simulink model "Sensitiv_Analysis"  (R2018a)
settings: Solver=ode4  StartTime=0.0  StopTime=40000  FixedStep=Ts  MaxStep=0.5  RelTol=1e-3  EnableMultiTasking=on
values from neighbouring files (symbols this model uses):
  Int_IC = [qti', 0 0, h0i(1:3)', 0 0, wr0, Vec0'*M0, Pec0']    [run.m]
  Kq1 = I22*ww^2 - 3*wo2*(I11-I33)    [run.m]
  Kq2 = 2*I22*zet*ww    [run.m]
  Kqi = 0.0005    [run.m]
  Kr1 = (0.1*I11*I33*zet^2/Hy0) - sqrt( ((0.01^zet^4*I11^2*I33^2)/Hy0^2)+(4*I11*I33*zet^2) )    [run.m]
  Kr2 = 0.05*Kr1    [run.m]
  Kr3 = 0.04*zet*(Kr2-Hy0) * sqrt(abs(Hy0/(I11*I33)))    [run.m]
  nt = 7    [run.m]    (also in runf.m)
  r2d = 180/pi    (= 57.2957795131)    [pl.m]    (also in pl2.m; run.m; plf.m; runf.m)
  Ts = 0.001    [run.m]    (also in runf.m = 0.0005)
undefined symbols (not defined in the file or in its folder): Aflx, Bflx, Cflx, den, Dflx, DiscIntNeverNeededParam, num, RW_Steering, Vehi_3B3W
libraries: simulink x3

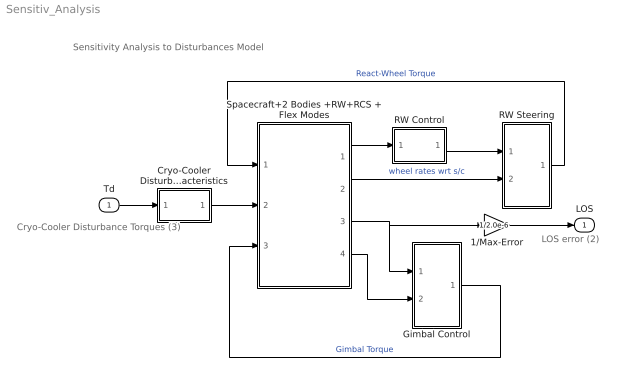
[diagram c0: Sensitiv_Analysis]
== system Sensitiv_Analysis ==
  note: Sensitivity Analysis to Disturbances Model
  note: LOS error (2)
  note: Cryo-Cooler Disturbance Torques (3)
  Td : Inport
  1/Max-Error : Gain  Gain=1/2.0e-6
  Cryo-Cooler Disturbance Characteristics : Subsystem
  Gimbal Control : Subsystem
  RW Control : Subsystem
  RW Steering : Subsystem
  Spacecraft+2 Bodies +RW+RCS + Flex Modes : Subsystem
  LOS : Outport
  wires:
  Spacecraft+2 Bodies +RW+RCS + Flex Modes/1(atti) -> RW Control/1(atti)
  Gimbal Control/1(GTrq) -> Spacecraft+2 Bodies +RW+RCS + Flex Modes/3(Tgimb)  "Gimbal Torque"
  RW Control/1(Tc) -> RW Steering/1(Trwc)
  Spacecraft+2 Bodies +RW+RCS + Flex Modes/2(Wrw) -> RW Steering/2(wr(1))  "wheel rates wrt s/c"
  RW Steering/1(Twi) -> Spacecraft+2 Bodies +RW+RCS + Flex Modes/1(Trw)  "React-Wheel Torque"
  Td/1 -> Cryo-Cooler Disturbance Characteristics/1(in)
  Spacecraft+2 Bodies +RW+RCS + Flex Modes/3(gimb) -> Gimbal Control/1(Gimb), 1/Max-Error/1
  Cryo-Cooler Disturbance Characteristics/1(ou) -> Spacecraft+2 Bodies +RW+RCS + Flex Modes/2(Tdist)
  1/Max-Error/1 -> LOS/1
  Spacecraft+2 Bodies +RW+RCS + Flex Modes/4(Gmb-dot) -> Gimbal Control/2(Grat)

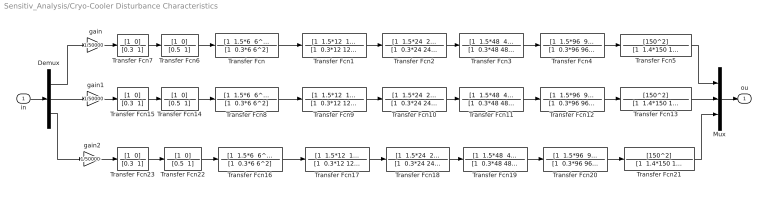
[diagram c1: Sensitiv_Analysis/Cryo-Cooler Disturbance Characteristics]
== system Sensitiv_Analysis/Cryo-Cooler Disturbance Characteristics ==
  in : Inport
  Demux : Demux  Outputs=3
  Mux : Mux  Inputs=3
  Transfer Fcn : TransferFcn  Numerator="[1  1.5*6  6^2]"  Denominator="[1  0.3*6 6^2]"
  Transfer Fcn1 : TransferFcn  Numerator="[1  1.5*12  12^2]"  Denominator="[1  0.3*12 12^2]"
  Transfer Fcn10 : TransferFcn  Numerator="[1  1.5*24  24^2]"  Denominator="[1  0.3*24 24^2]"
  Transfer Fcn11 : TransferFcn  Numerator="[1  1.5*48  48^2]"  Denominator="[1  0.3*48 48^2]"
  Transfer Fcn12 : TransferFcn  Numerator="[1  1.5*96  96^2]"  Denominator="[1  0.3*96 96^2]"
  Transfer Fcn13 : TransferFcn  Numerator=[150^2]  Denominator="[1  1.4*150 150^2]"
  Transfer Fcn14 : TransferFcn  Numerator="[1  0]"  Denominator="[0.5  1]"
  Transfer Fcn15 : TransferFcn  Numerator="[1  0]"  Denominator="[0.3  1]"
  Transfer Fcn16 : TransferFcn  Numerator="[1  1.5*6  6^2]"  Denominator="[1  0.3*6 6^2]"
  Transfer Fcn17 : TransferFcn  Numerator="[1  1.5*12  12^2]"  Denominator="[1  0.3*12 12^2]"
  Transfer Fcn18 : TransferFcn  Numerator="[1  1.5*24  24^2]"  Denominator="[1  0.3*24 24^2]"
  Transfer Fcn19 : TransferFcn  Numerator="[1  1.5*48  48^2]"  Denominator="[1  0.3*48 48^2]"
  Transfer Fcn2 : TransferFcn  Numerator="[1  1.5*24  24^2]"  Denominator="[1  0.3*24 24^2]"
  Transfer Fcn20 : TransferFcn  Numerator="[1  1.5*96  96^2]"  Denominator="[1  0.3*96 96^2]"
  Transfer Fcn21 : TransferFcn  Numerator=[150^2]  Denominator="[1  1.4*150 150^2]"
  Transfer Fcn22 : TransferFcn  Numerator="[1  0]"  Denominator="[0.5  1]"
  Transfer Fcn23 : TransferFcn  Numerator="[1  0]"  Denominator="[0.3  1]"
  Transfer Fcn3 : TransferFcn  Numerator="[1  1.5*48  48^2]"  Denominator="[1  0.3*48 48^2]"
  Transfer Fcn4 : TransferFcn  Numerator="[1  1.5*96  96^2]"  Denominator="[1  0.3*96 96^2]"
  Transfer Fcn5 : TransferFcn  Numerator=[150^2]  Denominator="[1  1.4*150 150^2]"
  Transfer Fcn6 : TransferFcn  Numerator="[1  0]"  Denominator="[0.5  1]"
  Transfer Fcn7 : TransferFcn  Numerator="[1  0]"  Denominator="[0.3  1]"
  Transfer Fcn8 : TransferFcn  Numerator="[1  1.5*6  6^2]"  Denominator="[1  0.3*6 6^2]"
  Transfer Fcn9 : TransferFcn  Numerator="[1  1.5*12  12^2]"  Denominator="[1  0.3*12 12^2]"
  gain : Gain  Gain=1/50000
  gain1 : Gain  Gain=1/50000
  gain2 : Gain  Gain=1/50000
  ou : Outport
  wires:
  Demux/1 -> gain/1
  Transfer Fcn/1 -> Transfer Fcn1/1
  Transfer Fcn1/1 -> Transfer Fcn2/1
  Transfer Fcn2/1 -> Transfer Fcn3/1
  Transfer Fcn3/1 -> Transfer Fcn4/1
  gain/1 -> Transfer Fcn7/1
  Transfer Fcn4/1 -> Transfer Fcn5/1
  Transfer Fcn5/1 -> Mux/1
  Transfer Fcn6/1 -> Transfer Fcn/1
  Transfer Fcn7/1 -> Transfer Fcn6/1
  Demux/2 -> gain1/1
  Transfer Fcn8/1 -> Transfer Fcn9/1
  Transfer Fcn9/1 -> Transfer Fcn10/1
  Transfer Fcn10/1 -> Transfer Fcn11/1
  Transfer Fcn11/1 -> Transfer Fcn12/1
  gain1/1 -> Transfer Fcn15/1
  Transfer Fcn12/1 -> Transfer Fcn13/1
  Transfer Fcn13/1 -> Mux/2
  Transfer Fcn14/1 -> Transfer Fcn8/1
  Transfer Fcn15/1 -> Transfer Fcn14/1
  Demux/3 -> gain2/1
  Transfer Fcn16/1 -> Transfer Fcn17/1
  Transfer Fcn17/1 -> Transfer Fcn18/1
  Transfer Fcn18/1 -> Transfer Fcn19/1
  Transfer Fcn19/1 -> Transfer Fcn20/1
  gain2/1 -> Transfer Fcn23/1
  Transfer Fcn20/1 -> Transfer Fcn21/1
  Transfer Fcn21/1 -> Mux/3
  Transfer Fcn22/1 -> Transfer Fcn16/1
  Transfer Fcn23/1 -> Transfer Fcn22/1
  Mux/1 -> ou/1
  in/1 -> Demux/1

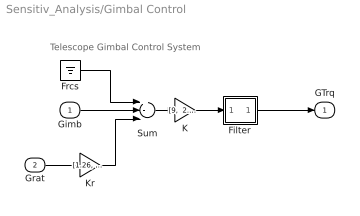
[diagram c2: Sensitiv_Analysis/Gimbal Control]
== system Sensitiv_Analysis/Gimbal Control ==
  note: Telescope Gimbal Control System
  Gimb : Inport
  Grat : Inport  Port=2
  Filter : Subsystem
  Frcs : Ground
  K : Gain  Gain="[9,  2.85]"
  Kr : Gain  Gain="[1.26,  1.14]"
  Sum : Sum  Inputs=+--
  GTrq : Outport
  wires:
  Filter/1(O) -> GTrq/1
  Sum/1 -> K/1
  Gimb/1 -> Sum/2
  Grat/1 -> Kr/1
  Kr/1 -> Sum/3
  Frcs/1 -> Sum/1
  K/1 -> Filter/1(I)

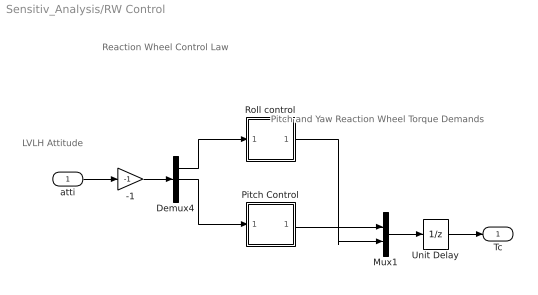
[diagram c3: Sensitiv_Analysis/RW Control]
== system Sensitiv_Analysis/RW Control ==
  note: Pitch and Yaw Reaction Wheel Torque Demands
  note: LVLH Attitude
  note: Reaction Wheel Control Law
  atti : Inport
  -1 : Gain  Gain=-1
  Demux4 : Demux  Outputs=3
  Mux1 : Mux  Inputs=2
  Pitch Control : Subsystem
  Roll control : Subsystem
  Unit Delay : UnitDelay  SampleTime=-1
  Tc : Outport
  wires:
  Demux4/1 -> Roll control/1(phi)
  Pitch Control/1(Tcy) -> Mux1/1
  Demux4/2 -> Pitch Control/1(the)
  atti/1 -> -1/1
  Roll control/1(Tcz) -> Mux1/2
  Mux1/1 -> Unit Delay/1
  -1/1 -> Demux4/1
  Unit Delay/1 -> Tc/1

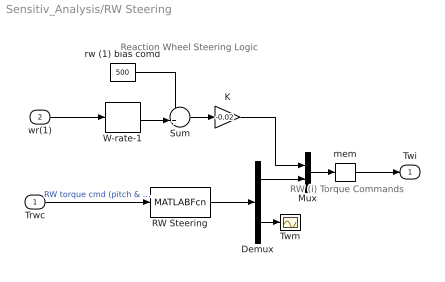
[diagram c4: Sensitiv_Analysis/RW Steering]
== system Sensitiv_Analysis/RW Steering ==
  note: Reaction Wheel Steering Logic
  note: RW (i) Torque Commands
  Trwc : Inport
  wr(1) : Inport  Port=2
  Demux : Demux  Outputs=[2, 1]
  K : Gain  Gain=-0.02
  Mux : Mux  Inputs=[1,2]
  RW Steering : MATLABFcn  MATLABFcn=RW_Steering( u(1:2) )  OutputDimensions=3
  Sum : Sum  Inputs=++|
  Twm : Scope
  W-rate-1 : Selector  InputPortWidth=3  IndexOptions=Index vector (dialog)  Indices=[1]  OutputSizes=1
  mem : Memory
  rw (1) bias comd : Constant  Value=500
  Twi : Outport
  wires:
  mem/1 -> Twi/1
  K/1 -> Mux/1
  W-rate-1/1 -> Sum/2
  rw (1) bias comd/1 -> Sum/1
  Sum/1 -> K/1
  wr(1)/1 -> W-rate-1/1
  Mux/1 -> mem/1
  Trwc/1 -> RW Steering/1  "RW torque cmd (pitch & yaw)"
  RW Steering/1 -> Demux/1
  Demux/1 -> Mux/2
  Demux/2 -> Twm/1

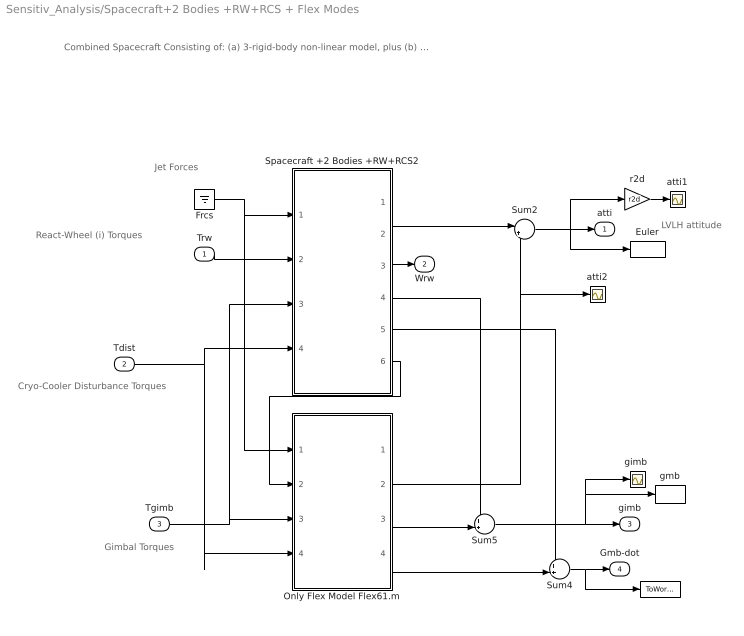
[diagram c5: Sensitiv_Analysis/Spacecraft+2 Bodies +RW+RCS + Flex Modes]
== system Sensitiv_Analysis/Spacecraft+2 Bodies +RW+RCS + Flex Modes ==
  note: LVLH attitude
  note: Combined Spacecraft Consisting of: (a) 3-rigid-body non-linear model, plus (b) a 61 flex modes state-space model
  note: Gimbal Torques
  note: Jet Forces
  note: React-Wheel (i) Torques
  note: Cryo-Cooler Disturbance Torques
  Trw : Inport
  Tdist : Inport  Port=2
  Tgimb : Inport  Port=3
  "   " : ToWorkspace  VariableName=Gimdot  SampleTime=-1
  Euler : ToWorkspace  VariableName=Euler  SampleTime=-1
  Frcs : Ground
  Only Flex Model Flex61.m : Subsystem
  Spacecraft +2 Bodies +RW+RCS2 : Subsystem
  Sum2 : Sum  Inputs=|++
  Sum4 : Sum  Inputs=++|
  Sum5 : Sum  Inputs=++|
  atti1 : Scope
  atti2 : Scope
  "gimb " : Scope
  gmb : ToWorkspace  VariableName=Gimb  SampleTime=-1
  r2d : Gain  Gain=r2d
  atti : Outport
  Wrw : Outport  Port=2
  gimb : Outport  Port=3
  Gmb-dot : Outport  Port=4
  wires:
  Frcs/1 -> Spacecraft +2 Bodies +RW+RCS2/1(Frcs), Only Flex Model Flex61.m/1(Fjets)
  Trw/1 -> Spacecraft +2 Bodies +RW+RCS2/2(Trw)
  Tgimb/1 -> Spacecraft +2 Bodies +RW+RCS2/3(Tgimb), Only Flex Model Flex61.m/3(Tgimb)
  Spacecraft +2 Bodies +RW+RCS2/2(att) -> Sum2/1
  Spacecraft +2 Bodies +RW+RCS2/4(gimb) -> Sum5/1
  Spacecraft +2 Bodies +RW+RCS2/5(Gmb-dot) -> Sum4/1
  Spacecraft +2 Bodies +RW+RCS2/3(W_rw) -> Wrw/1
  Sum2/1 -> atti/1, Euler/1, r2d/1
  Sum5/1 -> gimb/1, gmb/1, "gimb "/1
  Sum4/1 -> Gmb-dot/1, "   "/1
  r2d/1 -> atti1/1
  Only Flex Model Flex61.m/2(atti) -> atti2/1, Sum2/2
  Only Flex Model Flex61.m/3(gimb) -> Sum5/2
  Only Flex Model Flex61.m/4(Gmb-dot) -> Sum4/2
  Spacecraft +2 Bodies +RW+RCS2/6(Twb) -> Only Flex Model Flex61.m/2(Trwb)
  Tdist/1 -> Spacecraft +2 Bodies +RW+RCS2/4(Tdist), Only Flex Model Flex61.m/4(Tcryo)

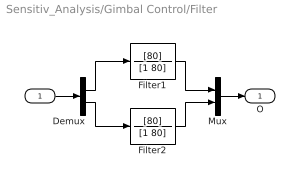
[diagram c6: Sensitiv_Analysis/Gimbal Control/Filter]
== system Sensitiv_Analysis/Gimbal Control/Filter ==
  I : Inport
  Demux : Demux  Outputs=2
  Filter1 : TransferFcn  Numerator=[80]  Denominator=[1 80]
  Filter2 : TransferFcn  Numerator=[80]  Denominator=[1 80]
  Mux : Mux  Inputs=2
  O : Outport
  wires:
  Filter1/1 -> Mux/1
  Filter2/1 -> Mux/2
  Demux/1 -> Filter1/1
  Demux/2 -> Filter2/1
  I/1 -> Demux/1
  Mux/1 -> O/1

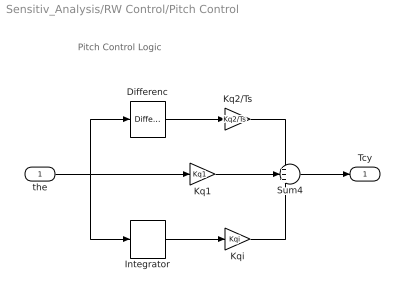
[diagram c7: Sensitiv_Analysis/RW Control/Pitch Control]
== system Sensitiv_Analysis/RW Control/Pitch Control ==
  note: Pitch Control Logic
  the : Inport
  Differenc : simulink/Discrete/Difference  ICPrevInput=-0.1757  InputProcessing=Inherited  OutMin=[]  OutMax=[]  OutDataType=sfix(16)  OutScaling=2^-10  DoSatur=off
  Integrator : DiscreteIntegrator  SampleTime=Ts  ICPrevOutput=DiscIntNeverNeededParam  ICPrevScaledInput=DiscIntNeverNeededParam
  Kq1 : Gain  Gain=Kq1
  Kq2/Ts : Gain  Gain=Kq2/Ts
  Kqi : Gain  Gain=Kqi
  Sum4 : Sum  Inputs=+++
  Tcy : Outport
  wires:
  Kq1/1 -> Sum4/2
  Sum4/1 -> Tcy/1
  the/1 -> Kq1/1, Differenc/1, Integrator/1
  Kqi/1 -> Sum4/3
  Integrator/1 -> Kqi/1
  Differenc/1 -> Kq2/Ts/1
  Kq2/Ts/1 -> Sum4/1

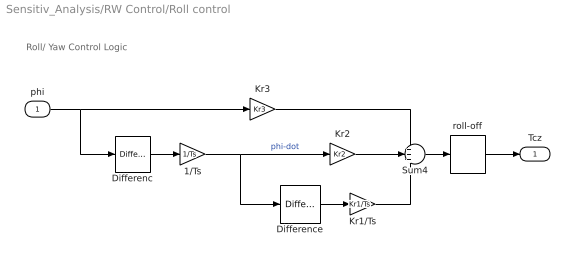
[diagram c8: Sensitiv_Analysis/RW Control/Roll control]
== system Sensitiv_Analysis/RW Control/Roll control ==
  note: Roll/ Yaw Control Logic
  phi : Inport
  1/Ts : Gain  Gain=1/Ts
  Differenc : simulink/Discrete/Difference  ICPrevInput=0  InputProcessing=Inherited  OutMin=[]  OutMax=[]  OutDataType=sfix(16)  OutScaling=2^-10  DoSatur=off
  Difference : simulink/Discrete/Difference  ICPrevInput=0.0  InputProcessing=Inherited  OutMin=[]  OutMax=[]  OutDataType=sfix(16)  OutScaling=2^-10  DoSatur=off
  Kr1/Ts : Gain  Gain=Kr1/Ts
  Kr2 : Gain  Gain=Kr2
  Kr3 : Gain  Gain=Kr3
  Sum4 : Sum  Inputs=+++
  roll-off : DiscreteTransferFcn  Numerator=[num]  Denominator=[den]  SampleTime=Ts
  Tcz : Outport
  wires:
  Kr3/1 -> Sum4/1
  Kr2/1 -> Sum4/2
  Kr1/Ts/1 -> Sum4/3
  phi/1 -> Kr3/1, Differenc/1
  Sum4/1 -> roll-off/1
  Difference/1 -> Kr1/Ts/1
  Differenc/1 -> 1/Ts/1
  1/Ts/1 -> Kr2/1, Difference/1  "phi-dot"
  roll-off/1 -> Tcz/1

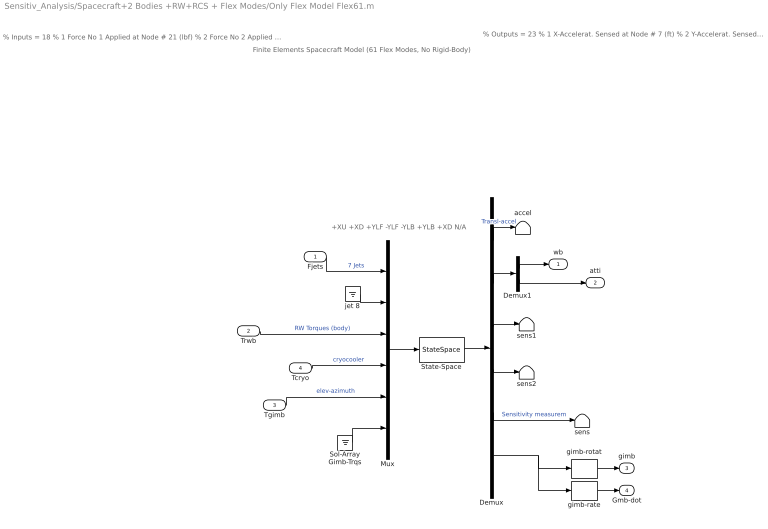
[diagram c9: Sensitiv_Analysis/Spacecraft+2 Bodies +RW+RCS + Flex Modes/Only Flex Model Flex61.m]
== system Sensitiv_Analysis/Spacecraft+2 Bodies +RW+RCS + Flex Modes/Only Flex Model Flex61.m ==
  note: +XU +XD +YLF -YLF -YLB +YLB +XD N/A
  note: % Outputs = 23 % 1 X-Accelerat. Sensed at Node # 7 (ft) % 2 Y-Accelerat. Sensed at Node # 7 (ft) % 3 X-Rot. Rate Sensed at Node # 6 (radian) % 4 Y-Rot. Rate Sensed at Node # 6 (radian) % 5 Z-Rot. Rate Sensed at Node # 6 (radian) % 6 X-Rotation Sensed at Node # 6 (radian) % 7 Y-Rotation Sensed at Node # 6 (radian) % 8 Z-Rotation Sensed at Node # 6 (radian) % 9 Y-Rotation Sensed at Node # 9 (radian) % 10 Z-Rotation Sensed at Node # 9 (radian) % 11 Y-Rotation Sensed at Node # 10 (radian) % 12 Z-Rotation Sensed at Node # 10 (radian) % 13 X-Rotation Sensed at Node # 11 (radian) % 14 Y-Rotation Sensed at Node # 12 (radian) % 15 Z-Rotation Sensed at Node # 13 (radian) % 16 Rotation Angle at Gimbal No 1 in (radians) % 17 Rotation Rate at Gimbal No 1 in (rad/sec) % 18 Rotation Angle at Gimbal No 2 in (radians) % 19 Rotation Rate at Gimbal No 2 in (rad/sec) % 20 Rotation Angle at Gimbal No 3 in (radians) % 21 Rotation Rate at Gimbal No 3 in (rad/sec) % 22 Rotation Angle at Gimbal No 4 in (radians) % 23 Rotation Rate at Gimbal No 4 in (rad/sec)
  note: % Inputs = 18 % 1 Force No 1 Applied at Node # 21 (lbf) % 2 Force No 2 Applied at Node # 22 (lbf) % 3 Force No 3 Applied at Node # 23 (lbf) % 4 Force No 4 Applied at Node # 24 (lbf) % 5 Force No 5 Applied at Node # 25 (lbf) % 6 Force No 6 Applied at Node # 26 (lbf) % 7 Force No 7 Applied at Node # 27 (lbf) % 8 Force No 8 Applied at Node # 28 (lbf) % 9 Torque No 1 Applied at Node # 17 (ft-lb) % 10 Torque No 2 Applied at Node # 18 (ft-lb) % 11 Torque No 3 Applied at Node # 19 (ft-lb) % 12 Torque No 4 Applied at Node # 8 (ft-lb) % 13 Torque No 5 Applied at Node # 8 (ft-lb) % 14 Torque No 6 Applied at Node # 8 (ft-lb) % 15 Control Torque at Gimbal No 1 in (ft-lb) % 16 Control Torque at Gimbal No 2 in (ft-lb) % 17 Control Torque at Gimbal No 3 in (ft-lb) % 18 Control Torque at Gimbal No 4 in (ft-lb)
  note: Finite Elements Spacecraft Model (61 Flex Modes, No Rigid-Body)
  Fjets : Inport
  Trwb : Inport  Port=2
  Tgimb : Inport  Port=3
  Tcryo : Inport  Port=4
  Demux : Demux  Outputs="[2, 6, 2,2,3,  8]"
  Demux1 : Demux  Outputs=[3, 3]
  Mux : Mux  Inputs=[7,1,3,3,2,2]
  Sol-Array Gimb-Trqs : Ground
  State-Space : StateSpace  A=Aflx  B=Bflx  C=Cflx  D=Dflx  InitialCondition=0
  accel : Terminator
  gimb-rate : Selector  InputPortWidth=8  IndexOptions=Index vector (dialog)  Indices=[2, 4]  OutputSizes=1
  gimb-rotat : Selector  InputPortWidth=8  IndexOptions=Index vector (dialog)  Indices=[1 3]  OutputSizes=1
  jet 8 : Ground
  sens : Terminator
  sens1 : Terminator
  sens2 : Terminator
  wb : Outport
  atti : Outport  Port=2
  gimb : Outport  Port=3
  Gmb-dot : Outport  Port=4
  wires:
  Demux1/2 -> atti/1
  Demux/5 -> sens/1  "Sensitivity measurem"
  Sol-Array Gimb-Trqs/1 -> Mux/6
  Tcryo/1 -> Mux/4  "cryocooler"
  Trwb/1 -> Mux/3  "RW Torques (body)"
  jet 8/1 -> Mux/2
  Fjets/1 -> Mux/1  "7 Jets"
  Mux/1 -> State-Space/1
  Demux1/1 -> wb/1
  Demux/2 -> Demux1/1
  State-Space/1 -> Demux/1
  Demux/1 -> accel/1  "Transl-accel"
  Tgimb/1 -> Mux/5  "elev-azimuth"
  Demux/6 -> gimb-rate/1, gimb-rotat/1
  Demux/3 -> sens1/1
  Demux/4 -> sens2/1
  gimb-rate/1 -> Gmb-dot/1
  gimb-rotat/1 -> gimb/1

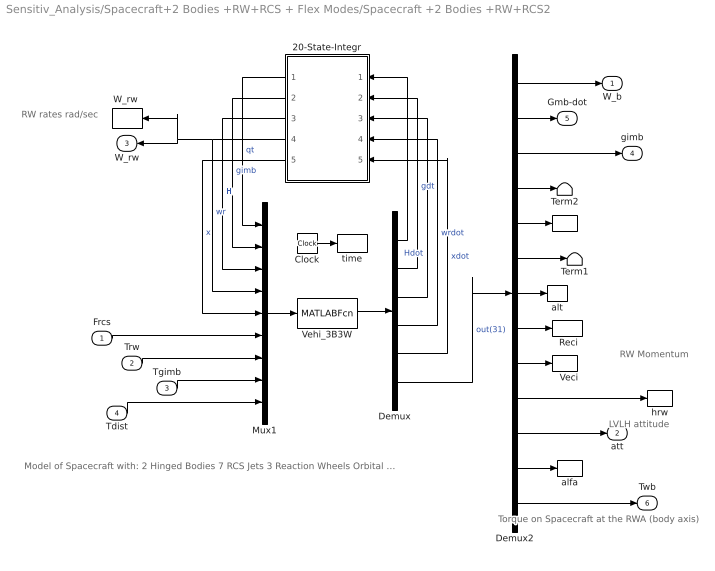
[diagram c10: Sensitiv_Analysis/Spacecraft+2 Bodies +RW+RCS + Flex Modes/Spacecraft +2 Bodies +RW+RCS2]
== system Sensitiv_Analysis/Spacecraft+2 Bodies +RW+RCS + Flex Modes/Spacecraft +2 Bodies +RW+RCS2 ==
  note: RW rates rad/sec
  note: RW Momentum
  note: Model of Spacecraft with: 2 Hinged Bodies 7 RCS Jets 3 Reaction Wheels Orbital Dynamics
  note: LVLH attitude
  note: Torque on Spacecraft at the RWA (body axis)
  Frcs : Inport
  Trw : Inport  Port=2
  Tgimb : Inport  Port=3
  Tdist : Inport  Port=4
  "    " : ToWorkspace  VariableName=hsys  SampleTime=-1
  "   Veci" : ToWorkspace  VariableName=Veci  SampleTime=-1
  "  Reci " : ToWorkspace  VariableName=Reci  SampleTime=-1
  20-State-Integr : Subsystem
  Clock : Clock
  Demux : Demux  Outputs="[4,2,5,3,6,  31]"
  Demux2 : Demux  Outputs=[3,2,2,1, 3,2, 1,3,3,3,3, 2,3]
  Mux1 : Mux  Inputs="[4,2,5,3,6,  nt,3,2,3]"
  Term1 : Terminator
  Term2 : Terminator
  Vehi_3B3W : MATLABFcn  MATLABFcn=Vehi_3B3W( u(1:20), u(21:20+nt), u(21+nt:23+nt), u(24+nt:25+nt), u(26+nt:28+nt) )  OutputDimensions=51
  "W_rw " : ToWorkspace  VariableName=W_rw  SampleTime=-1
  alfa : ToWorkspace  VariableName=alfa  SampleTime=-1
  alt : ToWorkspace  VariableName=alt  SampleTime=-1
  hrw : ToWorkspace  VariableName=hrw  SampleTime=-1
  time : ToWorkspace  VariableName=time  SampleTime=-1
  W_b : Outport
  att : Outport  Port=2
  W_rw : Outport  Port=3
  gimb : Outport  Port=4
  Gmb-dot : Outport  Port=5
  Twb : Outport  Port=6
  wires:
  Demux2/9 -> "   Veci"/1
  Vehi_3B3W/1 -> Demux/1
  20-State-Integr/1(qt) -> Mux1/1  "qt"
  20-State-Integr/2(gimb) -> Mux1/2  "gimb"
  20-State-Integr/3(H) -> Mux1/3  "H"
  20-State-Integr/4(wr) -> W_rw/1, "W_rw "/1, Mux1/4  "wr"
  20-State-Integr/5(x) -> Mux1/5  "x"
  Demux/6 -> Demux2/1  "out(31)"
  Demux/1 -> 20-State-Integr/1(qdot)
  Demux/2 -> 20-State-Integr/2(gmbdot)  "gdt"
  Demux/3 -> 20-State-Integr/3(Hdot)  "Hdot"
  Demux/4 -> 20-State-Integr/4(wrdor)  "wrdot"
  Demux/5 -> 20-State-Integr/5(xdot)  "xdot"
  Demux2/12 -> alfa/1
  Demux2/11 -> att/1
  Demux2/10 -> hrw/1
  Demux2/8 -> "  Reci "/1
  Demux2/7 -> alt/1
  Demux2/5 -> "    "/1
  Demux2/6 -> Term1/1
  Demux2/1 -> W_b/1
  Demux2/4 -> Term2/1
  Demux2/2 -> Gmb-dot/1
  Demux2/3 -> gimb/1
  Clock/1 -> time/1
  Tgimb/1 -> Mux1/8
  Trw/1 -> Mux1/7
  Mux1/1 -> Vehi_3B3W/1
  Demux2/13 -> Twb/1
  Frcs/1 -> Mux1/6
  Tdist/1 -> Mux1/9

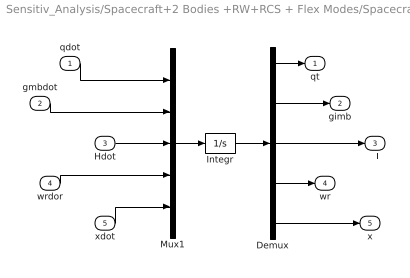
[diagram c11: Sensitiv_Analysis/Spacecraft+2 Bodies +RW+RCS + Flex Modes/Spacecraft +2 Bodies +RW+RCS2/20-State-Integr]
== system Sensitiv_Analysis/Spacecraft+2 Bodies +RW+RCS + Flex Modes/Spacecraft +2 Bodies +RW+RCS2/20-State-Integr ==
  qdot : Inport
  gmbdot : Inport  Port=2
  Hdot : Inport  Port=3
  wrdor : Inport  Port=4
  xdot : Inport  Port=5
  Demux : Demux  Outputs=[4,2,5,3,6]
  Integr : Integrator  InitialCondition=Int_IC
  Mux1 : Mux  Inputs=[4,2,5,3,6]
  qt : Outport
  gimb : Outport  Port=2
  H : Outport  Port=3
  wr : Outport  Port=4
  x : Outport  Port=5
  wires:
  Mux1/1 -> Integr/1
  Integr/1 -> Demux/1
  qdot/1 -> Mux1/1
  gmbdot/1 -> Mux1/2
  Hdot/1 -> Mux1/3
  wrdor/1 -> Mux1/4
  xdot/1 -> Mux1/5
  Demux/1 -> qt/1
  Demux/2 -> gimb/1
  Demux/3 -> H/1
  Demux/4 -> wr/1
  Demux/5 -> x/1
